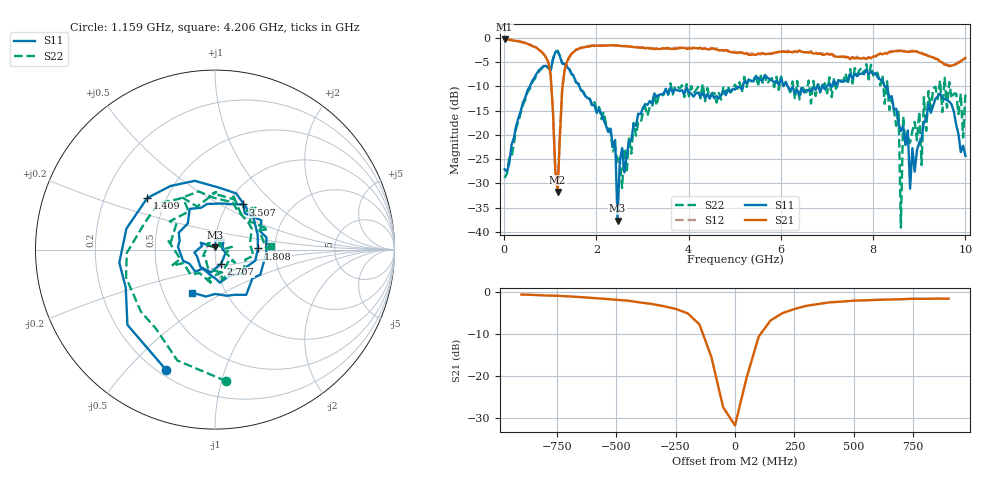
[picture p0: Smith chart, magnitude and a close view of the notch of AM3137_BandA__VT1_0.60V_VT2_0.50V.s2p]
! Date/Time: Tue, Nov 13, 2018 4:47 PM
! Network Analyzer: Agilent Technologies E8364B Rev: A.07.50.67
! Sweep from 0.010 to 10.000 GHz, 201 Points, Sweep Type: LIN
! Power Supply: 0.600 V, 0.000 A
# Hz S DB R 50
!freq MagS11 AngS11 MagS21 AngS21 MagS12 AngS12 MagS22 AngS22
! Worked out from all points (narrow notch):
!   201 points, 10 MHz to 10 GHz, reference 50 ohm
!   highest |S21| = -0.31 dB at 10 MHz (marker M1); lowest = -31.8 dB at 1.159 GHz (marker M2)
!   notch at M2: 28.9 dB deep, 157 MHz wide at half that depth
!   lowest |S11| = -37.7 dB at 2.458 GHz (marker M3), VSWR 1.03, Z = 50.2 + j1.29 ohm
!   |S11| at or under -10 dB: 1.63 GHz to 5.174 GHz (3.544 GHz wide, 104 % of centre); 6.147 GHz to 6.789 GHz (642.1 MHz wide, 9.93 % of centre); 8.303 GHz to end of sweep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
!   |S22| runs from -39.1 to -2.7 dB; largest |S21 - S12| = 0.029
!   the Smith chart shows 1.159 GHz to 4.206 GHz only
!   S11 on the Smith chart (normalised r, x): 1.159 GHz: 0.23, -0.65; 1.409 GHz: 0.39, +0.29; 1.808 GHz: 1.63, +0.02; 2.707 GHz: 1.06, -0.17; 3.507 GHz: 1.18, +0.65; 4.206 GHz: 0.70, -0.36
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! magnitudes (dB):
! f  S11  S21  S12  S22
! 10 MHz  -27.1  -0.3  -0.3  -28.9
! 959 MHz  -6.3  -5.1  -5.0  -6.0
! 1.159 GHz  -2.8  -31.8  -31.5  -2.7
! 1.259 GHz  -5.3  -10.6  -10.5  -5.2
! 1.409 GHz  -6.5  -4.1  -4.0  -6.2
! 1.708 GHz  -11.2  -2.0  -2.0  -11.0
! 1.808 GHz  -12.4  -1.8  -1.7  -12.4
! 2.408 GHz  -21.1  -1.6  -1.6  -22.5
! 2.458 GHz  -37.7  -1.6  -1.6  -25.9
! 2.707 GHz  -21.3  -1.8  -1.7  -20.4
! 3.357 GHz  -11.8  -2.3  -2.1  -11.6
! 3.507 GHz  -10.6  -2.2  -2.2  -10.5
! 4.206 GHz  -11.3  -2.2  -2.3  -10.1
! 5.005 GHz  -10.7  -3.1  -2.9  -9.7
! 6.703 GHz  -10.1  -3.3  -3.1  -8.9
! 8.352 GHz  -12.5  -2.9  -2.9  -14.9
! 8.551 GHz  -17.6  -2.8  -2.6  -15.0
! 8.601 GHz  -19.2  -2.7  -2.7  -39.1
! 8.651 GHz  -18.2  -2.8  -2.8  -16.2
! 8.801 GHz  -31.1  -2.9  -2.7  -21.6
! 9.451 GHz  -11.5  -4.9  -4.9  -8.8
! 10 GHz  -24.3  -4.2  -4.1  -11.7
